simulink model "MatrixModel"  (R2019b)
settings: Solver=ode45  StartTime=0.0  StopTime=10.0  RelTol=1e-3  EnableMultiTasking=on

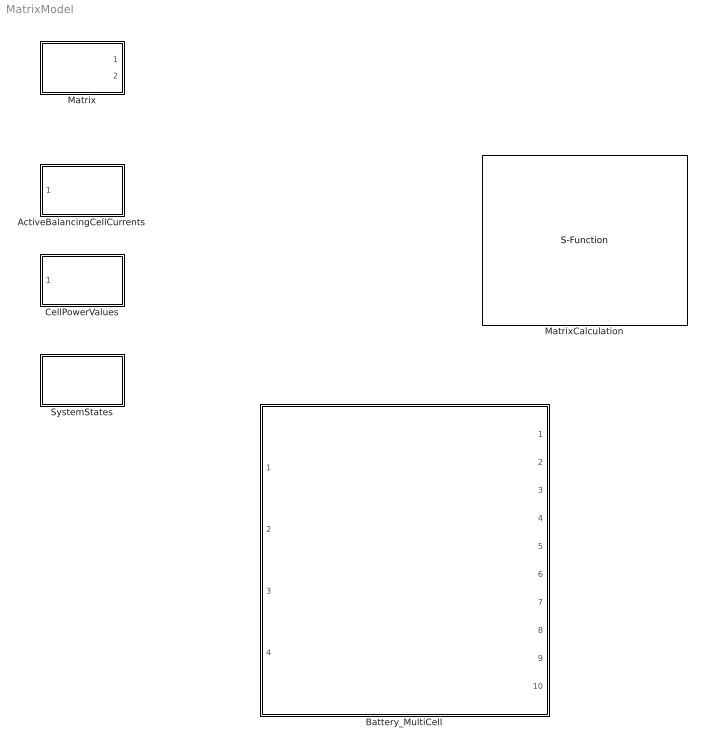
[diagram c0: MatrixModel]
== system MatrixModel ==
  ActiveBalancingCellCurrents : Subsystem
  Battery_MultiCell : Subsystem
  CellPowerValues : Subsystem
  Matrix : Subsystem
  MatrixCalculation : S-Function  FunctionName=MatrixCalculation  SFunctionDeploymentMode=off  EnableBusSupport=off
  SystemStates : Subsystem

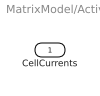
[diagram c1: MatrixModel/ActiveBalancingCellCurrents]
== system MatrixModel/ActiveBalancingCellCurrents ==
  CellCurrents : Inport

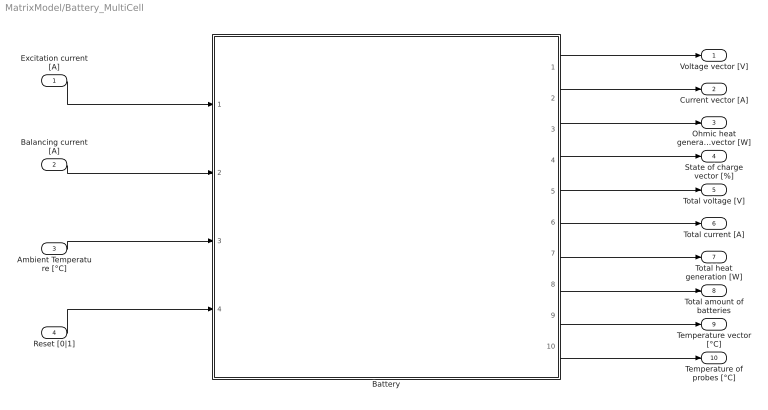
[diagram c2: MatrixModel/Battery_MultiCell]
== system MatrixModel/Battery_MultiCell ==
  Excitation current [A] : Inport
  Balancing current [A] : Inport  Port=2
  Ambient Temperature [°C] : Inport  Port=3
  Reset [0|1] : Inport  Port=4
  Battery : Subsystem
  Voltage vector [V] : Outport  VectorParamsAs1DForOutWhenUnconnected=off
  Current vector [A] : Outport  Port=2  VectorParamsAs1DForOutWhenUnconnected=off
  Ohmic heat generation vector [W] : Outport  Port=3  VectorParamsAs1DForOutWhenUnconnected=off
  State of charge vector [%] : Outport  Port=4  VectorParamsAs1DForOutWhenUnconnected=off
  Total voltage [V] : Outport  Port=5  VectorParamsAs1DForOutWhenUnconnected=off
  Total current [A] : Outport  Port=6  VectorParamsAs1DForOutWhenUnconnected=off
  Total heat generation [W] : Outport  Port=7  VectorParamsAs1DForOutWhenUnconnected=off
  Total amount of batteries : Outport  Port=8  VectorParamsAs1DForOutWhenUnconnected=off
  Temperature vector [°C] : Outport  Port=9  VectorParamsAs1DForOutWhenUnconnected=off
  Temperature of probes [°C] : Outport  Port=10  VectorParamsAs1DForOutWhenUnconnected=off
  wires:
  Excitation current [A]/1 -> Battery/1(ExcitationCurrent)
  Balancing current [A]/1 -> Battery/2(BalancingCurrent)
  Ambient Temperature [°C]/1 -> Battery/3(AmbientTemperature)
  Reset [0|1]/1 -> Battery/4(Reset)
  Battery/1(VoltageVector) -> Voltage vector [V]/1
  Battery/2(CurrentVector) -> Current vector [A]/1
  Battery/3(OhmicHeatGenerationVector) -> Ohmic heat generation vector [W]/1
  Battery/4(SocVector) -> State of charge vector [%]/1
  Battery/5(TotalVoltage) -> Total voltage [V]/1
  Battery/6(TotalCurrent) -> Total current [A]/1
  Battery/7(TotalHeatGeneration) -> Total heat generation [W]/1
  Battery/8(NumberOfBatteries) -> Total amount of batteries/1
  Battery/9(TemperatureVector) -> Temperature vector [°C]/1
  Battery/10(ProbeTemperatureVector) -> Temperature of probes [°C]/1

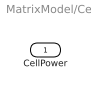
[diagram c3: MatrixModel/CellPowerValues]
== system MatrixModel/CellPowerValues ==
  CellPower : Inport

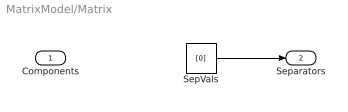
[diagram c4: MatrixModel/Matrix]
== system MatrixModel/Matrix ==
  SepVals : Constant  Value=[0]
  Components : Outport  VectorParamsAs1DForOutWhenUnconnected=off
  Separators : Outport  Port=2  VectorParamsAs1DForOutWhenUnconnected=off
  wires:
  SepVals/1 -> Separators/1

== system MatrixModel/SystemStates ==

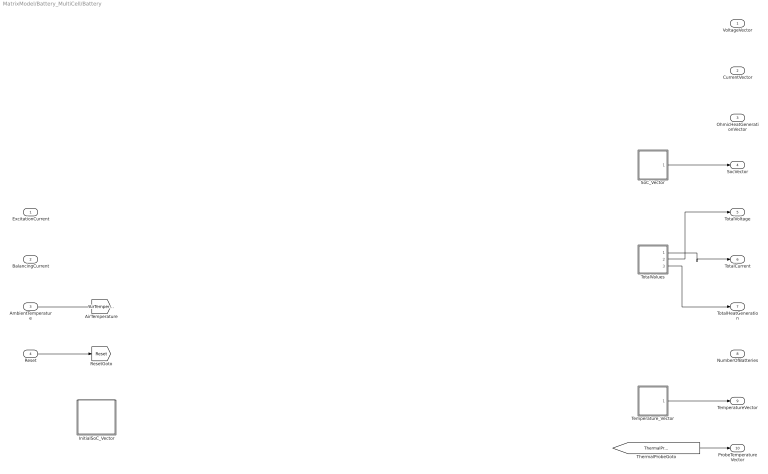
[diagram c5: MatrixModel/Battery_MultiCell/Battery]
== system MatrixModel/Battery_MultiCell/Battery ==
  ExcitationCurrent : Inport
  BalancingCurrent : Inport  Port=2
  AmbientTemperature : Inport  Port=3
  Reset : Inport  Port=4
  InitialSoC_Vector : Subsystem
  SoC_Vector : Subsystem
  Temperature_Vector : Subsystem
  TotalValues : Subsystem
  VoltageVector : Outport  VectorParamsAs1DForOutWhenUnconnected=off
  CurrentVector : Outport  Port=2  VectorParamsAs1DForOutWhenUnconnected=off
  OhmicHeatGenerationVector : Outport  Port=3  VectorParamsAs1DForOutWhenUnconnected=off
  SocVector : Outport  Port=4  VectorParamsAs1DForOutWhenUnconnected=off
  TotalVoltage : Outport  Port=5  VectorParamsAs1DForOutWhenUnconnected=off
  TotalCurrent : Outport  Port=6  VectorParamsAs1DForOutWhenUnconnected=off
  TotalHeatGeneration : Outport  Port=7  VectorParamsAs1DForOutWhenUnconnected=off
  NumberOfBatteries : Outport  Port=8  VectorParamsAs1DForOutWhenUnconnected=off
  TemperatureVector : Outport  Port=9  VectorParamsAs1DForOutWhenUnconnected=off
  ProbeTemperatureVector : Outport  Port=10  VectorParamsAs1DForOutWhenUnconnected=off
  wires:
  Temperature_Vector/1(TemperatureVector) -> TemperatureVector/1
  SoC_Vector/1(SocVector) -> SocVector/1
  TotalValues/1(Current) -> TotalCurrent/1
  TotalValues/3(Power) -> TotalHeatGeneration/1
  TotalValues/2(Voltage) -> TotalVoltage/1
  AmbientTemperature/1 -> [AirTemperature]
  Reset/1 -> [Reset]
  [ThermalProbeTemperatures] -> ProbeTemperatureVector/1

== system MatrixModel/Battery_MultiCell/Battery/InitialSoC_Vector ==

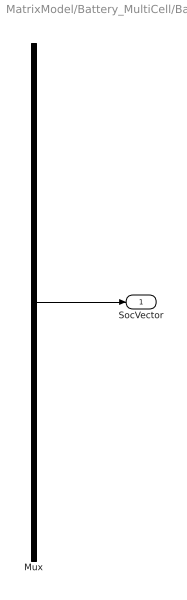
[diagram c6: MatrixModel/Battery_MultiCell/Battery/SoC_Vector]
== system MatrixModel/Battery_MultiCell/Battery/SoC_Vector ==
  Mux : Mux  Inputs=3
  SocVector : Outport  VectorParamsAs1DForOutWhenUnconnected=off
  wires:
  Mux/1 -> SocVector/1

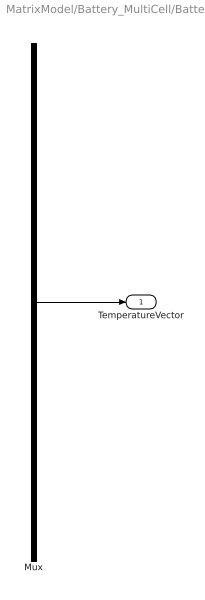
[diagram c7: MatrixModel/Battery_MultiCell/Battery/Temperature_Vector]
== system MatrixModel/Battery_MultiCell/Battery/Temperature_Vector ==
  Mux : Mux  Inputs=3
  TemperatureVector : Outport  VectorParamsAs1DForOutWhenUnconnected=off
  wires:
  Mux/1 -> TemperatureVector/1

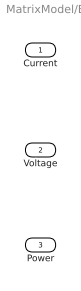
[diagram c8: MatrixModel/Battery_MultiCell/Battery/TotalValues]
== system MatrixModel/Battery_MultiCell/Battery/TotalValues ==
  Current : Outport  VectorParamsAs1DForOutWhenUnconnected=off
  Voltage : Outport  Port=2  VectorParamsAs1DForOutWhenUnconnected=off
  Power : Outport  Port=3  VectorParamsAs1DForOutWhenUnconnected=off
